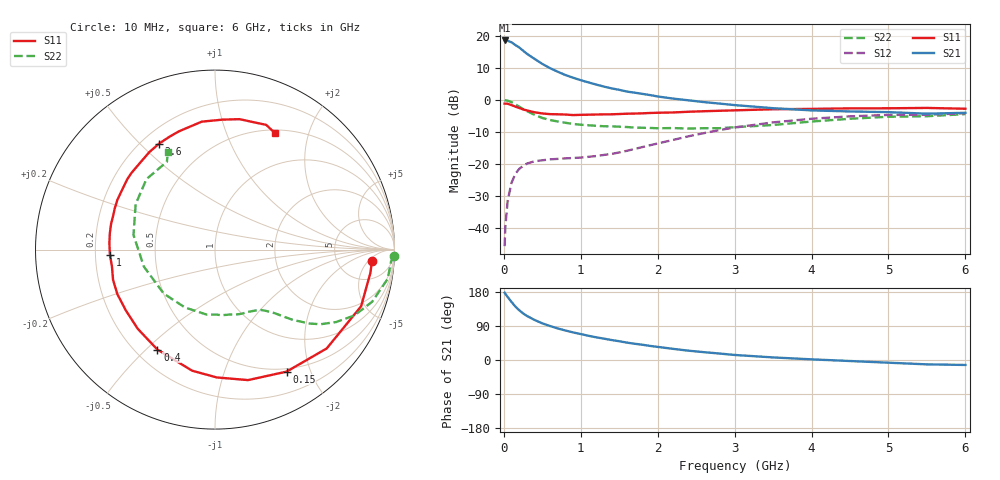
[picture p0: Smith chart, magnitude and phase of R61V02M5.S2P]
! SIEMENS Small Signal Semiconductors
! BFR193
! Si NPN RF Bipolar Junction Transistor in SOT23
! VCE = 1 V  IC = 2.5 mA
! Common Emitter S-Parameters:  May  1996
# GHz  S  MA  R  50
!  f  S11  S21  S12  S22
! GHz  MAG  ANG  MAG  ANG  MAG  ANG  MAG  ANG
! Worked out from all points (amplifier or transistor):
!   36 points, 10 MHz to 6 GHz, reference 50 ohm
!   highest |S21| = 18.5 dB at 10 MHz (marker M1)
!   |S21| within 3 dB of that: start of sweep to 241.4 MHz
!   unconditionally stable (mu >= 1): 1.076 GHz to 2.206 GHz; 5.645 GHz to end of sweep
!   at 250 MHz: K = 0.28, MSG = 17.9 dB, |S12| = -20.5 dB
!   at 1.4 GHz: K = 1.12, MAG = 8.1 dB, |S12| = -16.8 dB
!   at 6 GHz: K = 1.00, MAG = -0.2 dB, |S12| = -4.1 dB
!   S11 on the Smith chart (normalised r, x): 10 MHz: 12, -7; 150 MHz: 0.46, -1.65; 400 MHz: 0.29, -0.54; 1 GHz: 0.26, -0.02; 2.6 GHz: 0.27, +0.57; 6 GHz: 0.55, +1.51
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0.01  0.8771 -4.3  8.43 177.5  0.0053 88.8  0.9954 -1.9
0.02  0.8753 -8.6  8.273 174.3  0.0108 86.1  0.9834 -3.8
0.05  0.8732 -21.2  8.32 166.1  0.0271 78.3  0.9761 -9.6
0.1  0.8311 -41.5  7.891 153.2  0.0513 68.2  0.9222 -18.4
0.15  0.7882 -59.6  7.157 141.0  0.0709 59.4  0.8586 -25.3
0.2  0.75 -75.8  6.562 131.3  0.0845 52.5  0.7861 -30.9
0.25  0.7124 -89.2  5.851 123.0  0.0942 46.8  0.7211 -35.2
0.3  0.6866 -100.7  5.231 116.3  0.1023 43.0  0.671 -37.9
0.4  0.6427 -120.0  4.35 105.6  0.1112 37.4  0.5864 -42.0
0.5  0.6163 -134.3  3.639 96.7  0.1151 34.5  0.5242 -44.8
0.6  0.6014 -145.6  3.127 89.7  0.1189 33.1  0.4874 -46.7
0.7  0.598 -155.4  2.751 83.3  0.121 32.8  0.4623 -48.6
0.8  0.5926 -163.4  2.441 77.9  0.1231 33.2  0.4415 -50.5
1  0.5862 -177.2  2.029 68.4  0.1268 37.0  0.4115 -55.0
1.1  0.5896 176.5  1.875 63.9  0.1303 39.1  0.4033 -57.8
1.6  0.6105 152.9  1.35 45.9  0.1616 50.1  0.3791 -73.1
2.2  0.6388 130.8  1.05 29.4  0.2387 55.1  0.3652 -97.2
2.6  0.6676 117.9  0.926 20.7  0.3043 52.4  0.3632 -117.2
3.5  0.7167 95.9  0.744 6.8  0.4475 37.7  0.4076 -166.6
4.5  0.7396 79.3  0.662 -2.7  0.5559 18.8  0.5094 150.2
5.5  0.7512 67.7  0.611 -11.5  0.5883 1.6  0.5579 118.7
6  0.7294 62.5  0.631 -13.1  0.6206 -3.3  0.6017 115.9
